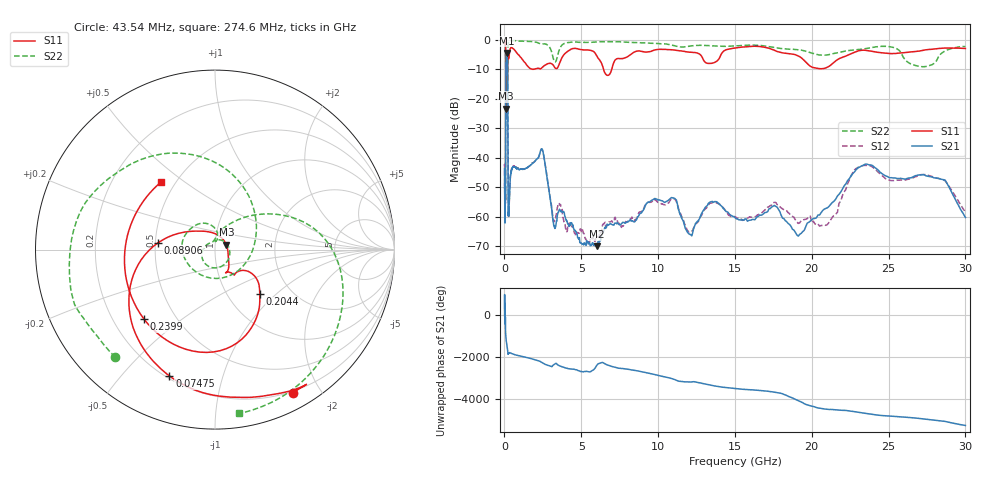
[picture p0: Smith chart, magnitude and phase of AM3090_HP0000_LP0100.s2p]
! Date/Time: Thu, Feb 28, 2019 1:52 PM
! Network Analyzer: Agilent Technologies E8364B Rev: A.07.50.67
! Sweep from 0.010 to 30.000 GHz, 1601 Points, Sweep Type: LOG
! Power Supply: 5.023 V, 0.002 A
# Hz S DB R 50
!freq MagS11 AngS11 MagS21 AngS21 MagS12 AngS12 MagS22 AngS22
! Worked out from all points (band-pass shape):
!   1601 points, 10 MHz to 30 GHz, reference 50 ohm
!   highest |S21| = -4.36 dB at 141.1 MHz (marker M1); lowest = -70.0 dB at 6.019 GHz (marker M2)
!   |S21| within 3 dB of the highest: 98.58 MHz to 196.1 MHz (97.55 MHz wide, 66.2 % of centre)
!   lowest |S11| = -23.3 dB at 97.46 MHz (marker M3), VSWR 1.15, Z = 56.7 + j3.07 ohm
!   |S11| at or under -10 dB: 89.15 MHz to 199.5 MHz (110.3 MHz wide, 76.5 % of centre); 6.455 GHz to 6.98 GHz (524.9 MHz wide, 7.81 % of centre)
!   |S22| runs from -27.0 to -0.1 dB; largest |S21 - S12| = 0.014
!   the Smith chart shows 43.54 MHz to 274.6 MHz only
!   S11 on the Smith chart (normalised r, x): 43.54 MHz: 0.18, -1.67; 74.75 MHz: 0.21, -0.68; 89.06 MHz: 0.51, +0.04; 204.4 MHz: 1.40, -0.80; 239.9 MHz: 0.33, -0.37; 274.6 MHz: 0.42, +0.41
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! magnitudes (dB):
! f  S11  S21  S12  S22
! 10 MHz  -0.2  -43.7  -42.8  -0.5
! 38.04 MHz  -0.5  -61.5  -59.1  -1.4
! 43.54 MHz  -0.8  -59.3  -59.4  -1.7
! 74.75 MHz  -2.5  -44.2  -43.9  -4.6
! 89.06 MHz  -9.9  -15.4  -15.4  -15.6
! 97.46 MHz  -23.3  -7.8  -7.7  -14.6
! 141.1 MHz  -15.6  -4.4  -4.3  -22.7
! 144.7 MHz  -15.4  -4.4  -4.3  -21.9
! 184.9 MHz  -14.0  -5.8  -5.8  -27.0
! 204.4 MHz  -9.1  -9.8  -9.8  -14.9
! 239.9 MHz  -5.1  -55.4  -54.2  -1.7
! 274.6 MHz  -6.3  -58.7  -59.6  -0.7
! 550.5 MHz  -2.9  -43.0  -42.9  -0.2
! 2.084 GHz  -9.7  -40.5  -40.6  -0.8
! 2.507 GHz  -9.1  -37.9  -38.0  -1.3
! 3.236 GHz  -9.0  -63.0  -61.7  -7.1
! 6.019 GHz  -5.5  -70.0  -66.8  -0.7
! 7.926 GHz  -5.9  -61.9  -61.9  -0.8
! 10.76 GHz  -3.3  -53.9  -54.7  -1.6
! 19.22 GHz  -5.6  -65.9  -62.0  -3.4
! 23.59 GHz  -3.6  -42.1  -42.5  -2.8
! 30 GHz  -2.9  -60.2  -58.4  -2.2
